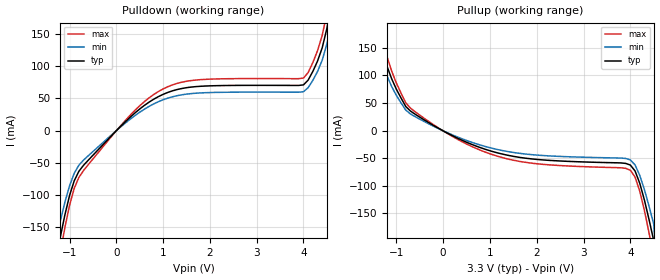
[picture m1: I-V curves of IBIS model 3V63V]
[IBIS Ver]   2.1
[File name]   55201_3.ibs
[File Rev]   2.0
[Date]   02/17/2000
[Source]   ICS MicroClock Applications Engineering 2
[Disclaimer] This information is for modeling purposes only, and is
(C) Copyright Integrated Circuit Systems, Inc. 1997-2001
   All rights reserved
ICS hereby grants the user of this IBIS model a non-exclusive,
nontransferable license to use this IBIS model under the following terms.
Before using this IBIS model, the user should read this license.
If the user does not accept these terms,  the IBIS model should be
returned to ICS within 30 days.
   The user is granted this license only to use the IBIS model and
is not granted rights to sell, load, rent, lease or license the IBIS
model in whole or in part, or in modified form to anyone other than
user. User may modify the IBIS model to suit its specific
applications but rights to derivative works and such modifications
shall belong to ICS.
   This IBIS model is provided on an "AS IS" basis and ICS makes
absolutely no warranty with respect to the information contained
herein. ICS DISCLAIMS AND CUSTOMER WAIVES ALL WARRANTIES, EXPRESS
OR IMPLIED, INCLUDING WARRANTIES OF MERCHANTABILITY OR FITNESS FOR
A PARTICULAR PURPOSE. The entire risk as to quality and performance
is with the Customer. ACCORDINGLY, IN NO EVENT SHALL THE COMPANY BE
LIABLE FOR ANY DAMAGES, WHETHER IN CONTRACT OR TORT,INCLUDING ANY
LOST PROFITS OR OTHER INCIDENTAL, CONSEQUENTIAL, EXEMPLARY, OR
PUNITIVE DAMAGES ARISING OUT OF THE USE OR APPLICATION OF THE IBIS
model provided in this package. Further, ICS reserves the right to
make changes without notice to any product herein to improve
reliability, function, or design. ICS does not convey any license
under patent rights or any other intellectual property rights,
including those of third parties.
   ICS is not obligated to provide maintenance or support
for the licensed IBIS model.
[Component]   ICS552-01
[Manufacturer] Integrated Circuit Systems Inc.
[Package]
|   typ   min   max
R_pkg   40m   35m   45m
L_pkg   1.65nH   1.35nH   1.95nH
C_pkg   0.24pF   0.14pF   0.34pF
[pin]   signal_name   model_name   R_pin   L_pin   C_pin
   7   CLK1(QA1)   3V63V
   8   CLK2(QA2)   3V63V
   9   CLK3(QA3)   3V63V
   10   CLK4(QA4)   3V63V
   12   CLK5(QB1)   3V63V
   13   CLK6(QB2)   3V63V
   17   CLK7(QB3)   3V63V
   18   CLK8(QB4)   3V63V
| Models and submodels in the file (1): 3V63V (Output)
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|   ICS552-01 3.3V Clock Drive Model
| This model is suitable for all output pins on the
| ICS552-01
[Model]   3V63V
Model_type   Output
Polarity   Non-Inverting
|   typ   min   max
C_comp   5pF   4pF   6pF
|   typ   min   max
[Voltage range]  3.3V   3.15V   3.45V
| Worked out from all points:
|   slope of the pulldown table from 0 to 0.495 V, typ, clamps not added: 14.9 ohm
|   slope of the pullup table from 0 to 0.495 V, typ, clamps not added: 24.2 ohm
[pulldown]
|Voltage I (typ)   I (min)   I (max)
-3.3V     -3A        -3A        -3A
-1.3V     -199.9mA   -169.9mA   -229.9mA
-1.2V     -166.1mA   -141.2mA   -191mA
-1.1V     -131mA     -111.3mA   -150.6mA
-800mV    -63.14mA   -53.66mA   -72.61mA
400mV     27.29mA    23.2mA     31.39mA
1.1V      58.96mA    50.11mA    67.8mA
4V        70.65mA    60.05mA    81.25mA
4.3V      107.5mA    91.34mA    123.6mA
4.5V      157.8mA    134.1mA    181.5mA
4.6V      195.8mA    166.4mA    225.2mA
6.6V      3A         3A         3A
[pullup]
|Voltage I (typ)   I (min)   I (max)
-3.3V     3A         3A         3A
-1.4V     190.5mA    161.9mA    219.1mA
-1.3V     149.2mA    126.8mA    171.6mA
-1.2V     116.4mA    98.91mA    133.8mA
-800mV    43.62mA    37.08mA    50.17mA
400mV     -17.51mA   -14.88mA   -20.14mA
1.6V      -48.26mA   -41.02mA   -55.49mA
4V        -62.64mA   -53.25mA   -72.04mA
4.2V      -95.46mA   -81.14mA   -109.8mA
4.4V      -161.7mA   -137.4mA   -185.9mA
4.5V      -199.9mA   -169.9mA   -229.9mA
6.6V      -3A        -3A        -3A
[Ramp]
|   typ   min   max
dV/dt_r   1.31/0.41n   1.24/0.45n   1.37/0.37n
dV/dt_f   1.54/0.34n   1.46/0.38n   1.62/0.31n
